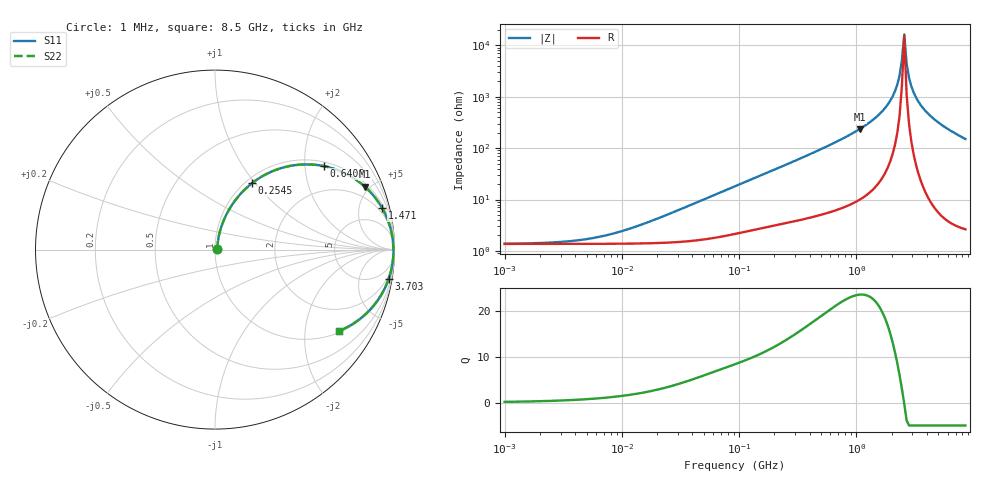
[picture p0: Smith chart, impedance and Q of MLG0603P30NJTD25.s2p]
! S-Parameter Data Generated by TDK Corporation
! Copyright(C) 2025 TDK Corporation.
! All Rights Reserved.
! TDK P/N: MLG0603P30NJTD25 (SMD / SMT Inductor (Coil))
! Property: L=30nH at 500MHz
! Size(LxWxT): 0.6x0.3x0.3mm
! Model Type: s2p (Touchstone File Format Version 1.0)
! Frequency: DC=Yes Start=1MHz Stop=8500MHz 198points Log-sweep
! Model Generated on Feb. 6, 2025
! Terms and conditions regarding TDK Simulation Models:
! 1)This simulation model is being provided solely for informational
!  purposes. Please refer to the specifications of the products in
!  terms of detailed characteristics of such products.
! 2)In no event shall TDK Corporation of any of its subsidiaries be
!  liable for any loss or damage arising, directly or indirectly,
!  from any information contained in this simulation model, including,
!  but not limited to loss or damages arising from any inaccuracies,
!  omissions or errors in connection with such information.
! 3)Any and all copyrights on this simulation model are owned by
!  TDK Corporation.  Duplication or redistribution of this simulation
!  model without prior written permission from TDK Corporation
!  is prohibited.
! 4)This simulation model is subject to any modification or change
!  without any prior notice.
! 5)Neither TDK Corporation nor any of its subsidiaries shall make any
!  warranty, express or implied, including but not limited to the
!  correctness, implied warranties of merchantability and fitness for
!  a particular purpose with respect to this simulation models.
! 6)The use of this simulation model shall be deemed to have consented
!  to the terms and conditions hereof.
! Port Assignments:
!  1 ---@@@--- 2
! Applicable Conditions:
!  Temperature = 25 degC
!  DC Bias Current = 0 A
!  Small Signal Operation
# Hz S MA R 50
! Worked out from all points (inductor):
!   197 points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, 1 MHz to 8.5 GHz, reference 50 ohm
!   read as one part in series: L = 31.7 nH near 22.04 MHz
!   highest Q = 23.6 at 1.065 GHz (marker M1), where L = 34.9 nH
!   self-resonance near 2.444 GHz
!   S11 on the Smith chart (normalised r, x): 1 MHz: 1.03, +0.00; 254.5 MHz: 1.07, +0.96; 640.8 MHz: 1.12, +2.50; 1.471 GHz: 1.36, +7.95; 3.703 GHz: 1, -12; 8.5 GHz: 1.05, -3.00
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1000000  0.01366 8.2  0.9865 -0.1  0.9865 -0.1  0.01366 8.2
4587603  0.01629 33.3  0.9864 -0.5  0.9864 -0.5  0.01629 33.3
9168677  0.02265 52.0  0.9862 -1.0  0.9862 -1.0  0.02265 52.0
2.10461e7  0.04373 68.8  0.985 -2.4  0.985 -2.4  0.04373 68.8
9.219544e7  0.1741 73.2  0.9643 -10.0  0.9643 -10.0  0.1741 73.2
1.604302e8  0.2864 68.2  0.9323 -16.6  0.9323 -16.6  0.2864 68.2
2.545462e8  0.422 60.9  0.8765 -24.9  0.8765 -24.9  0.422 60.9
4.229561e8  0.6092 49.3  0.7591 -37.5  0.7591 -37.5  0.6092 49.3
6.408078e8  0.7633 37.6  0.6106 -49.7  0.6106 -49.7  0.7633 37.6
1.064771e9  0.9055 22.8  0.3876 -64.8  0.3876 -64.8  0.9055 22.8
1.470933e9  0.9595 13.9  0.2412 -73.4  0.2412 -73.4  0.9595 13.9
1.940355e9  0.9851 6.8  0.1188 -79.4  0.1188 -79.4  0.9851 6.8
2.128028e9  0.9899 4.5  0.07867 -80.4  0.07867 -80.4  0.9899 4.5
2.333852e9  0.9929 2.2  0.03879 -78.3  0.03879 -78.3  0.9929 2.2
2.444114e9  0.9937 1.0  0.01923 -70.4  0.01923 -70.4  0.9937 1.0
2.559585e9  0.9941 -0.1  0.006146 17.0  0.006146 17.0  0.9941 -0.1
2.680511e9  0.9941 -1.3  0.02259 74.3  0.02259 74.3  0.9941 -1.3
2.80715e9  0.9937 -2.4  0.04232 80.2  0.04232 80.2  0.9937 -2.4
3.07866e9  0.9915 -4.7  0.08251 81.7  0.08251 81.7  0.9915 -4.7
3.703002e9  0.9816 -9.5  0.1643 78.9  0.1643 78.9  0.9816 -9.5
5.115526e9  0.9446 -18.2  0.3123 70.8  0.3123 70.8  0.9446 -18.2
8.5e9  0.8257 -33.3  0.5497 55.7  0.5497 55.7  0.8257 -33.3
